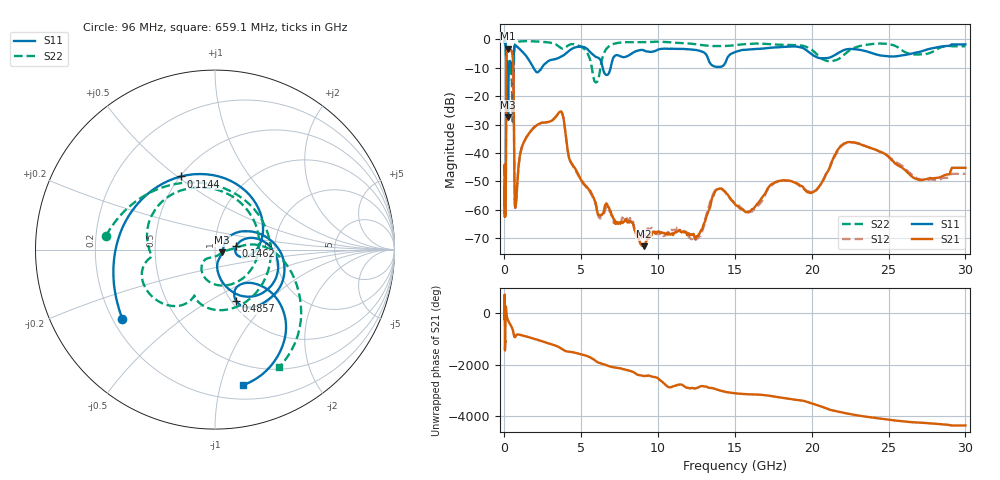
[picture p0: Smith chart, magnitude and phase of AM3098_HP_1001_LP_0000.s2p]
! Date/Time: Thu, Feb 28, 2019 8:40 AM
! Network Analyzer: Agilent Technologies E8364B Rev: A.07.50.67
! Sweep from 0.010 to 30.000 GHz, 1601 Points, Sweep Type: LOG
! Power Supply: 5.023 V, 0.002 A
# Hz S DB R 50
!freq MagS11 AngS11 MagS21 AngS21 MagS12 AngS12 MagS22 AngS22
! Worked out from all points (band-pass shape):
!   1601 points, 10 MHz to 30 GHz, reference 50 ohm
!   highest |S21| = -3.25 dB at 237.5 MHz (marker M1); lowest = -72.9 dB at 9.072 GHz (marker M2)
!   |S21| within 3 dB of the highest: 129.4 MHz to 537.9 MHz (408.5 MHz wide, 122 % of centre)
!   lowest |S11| = -27.5 dB at 237.5 MHz (marker M3), VSWR 1.09, Z = 54.1 - j1.68 ohm
!   |S11| at or under -10 dB: 198.7 MHz to 291.5 MHz (92.84 MHz wide, 37.9 % of centre); 1.889 GHz to 2.426 GHz (537.2 MHz wide, 24.9 % of centre); 6.392 GHz to 6.911 GHz (518.8 MHz wide, 7.8 % of centre)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
!   |S22| runs from -29.0 to -0.5 dB; largest |S21 - S12| = 0.012
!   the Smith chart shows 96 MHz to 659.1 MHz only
!   S11 on the Smith chart (normalised r, x): 96 MHz: 0.24, -0.32; 114.4 MHz: 0.50, +0.51; 146.2 MHz: 1.27, +0.05; 485.7 MHz: 1.05, -0.67; 659.1 MHz: 0.31, -1.17
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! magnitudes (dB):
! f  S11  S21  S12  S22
! 10 MHz  -0.3  -46.8  -45.1  -0.6
! 38.04 MHz  -0.5  -61.6  -60.2  -0.7
! 85.57 MHz  -2.5  -55.0  -57.7  -2.7
! 96 MHz  -3.8  -45.4  -43.6  -4.3
! 114.4 MHz  -6.9  -16.6  -16.6  -10.2
! 144.7 MHz  -18.8  -4.4  -4.3  -10.6
! 146.2 MHz  -18.4  -4.3  -4.3  -10.3
! 190.6 MHz  -9.0  -3.7  -3.7  -7.2
! 237.5 MHz  -27.5  -3.2  -3.2  -9.0
! 302 MHz  -9.1  -3.5  -3.4  -8.0
! 485.7 MHz  -10.2  -4.4  -4.4  -15.4
! 550.5 MHz  -11.2  -7.2  -7.2  -27.4
! 659.1 MHz  -2.2  -54.1  -54.6  -2.5
! 2.084 GHz  -11.5  -30.3  -30.3  -0.7
! 3.686 GHz  -6.1  -25.5  -25.5  -3.1
! 5.959 GHz  -6.2  -58.2  -58.7  -15.2
! 7.926 GHz  -6.1  -63.7  -63.1  -1.0
! 9.072 GHz  -3.8  -72.9  -69.0  -0.9
! 12.43 GHz  -3.7  -70.4  -70.4  -1.6
! 13.88 GHz  -9.7  -52.8  -52.7  -2.3
! 22.67 GHz  -3.4  -36.3  -36.3  -3.2
! 30 GHz  -1.7  -45.3  -47.4  -2.4
